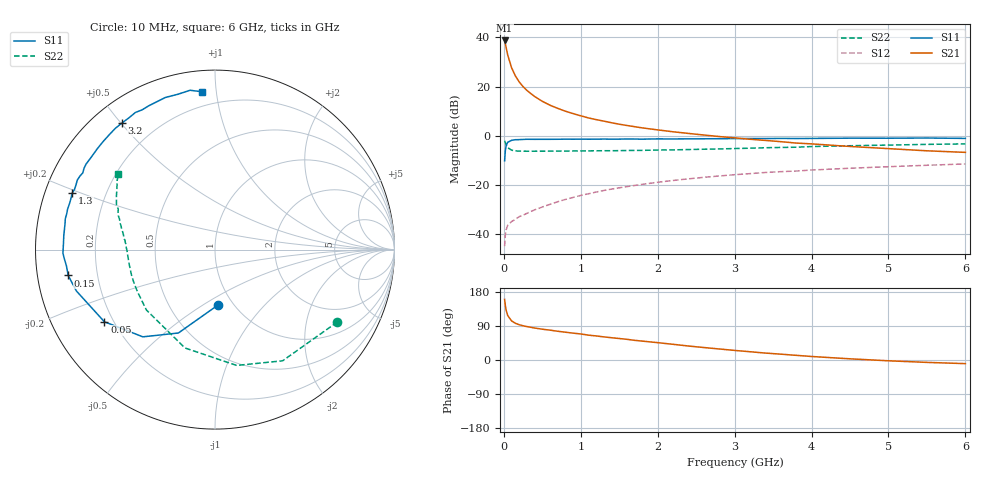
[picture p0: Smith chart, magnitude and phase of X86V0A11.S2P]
! SIEMENS Small Signal Semiconductors
! BFP136W
! Si NPN RF Bipolar Junction Transistor in SOT343
! VCE = 6 V  IC = 110 mA
! Common Emitter S-Parameters:  September  1994
# GHz  S  MA  R  50
!  f  S11  S21  S12  S22
! GHz  MAG  ANG  MAG  ANG  MAG  ANG  MAG  ANG
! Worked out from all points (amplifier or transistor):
!   40 points, 10 MHz to 6 GHz, reference 50 ohm
!   highest |S21| = 38.7 dB at 10 MHz (marker M1)
!   |S21| within 3 dB of that: start of sweep to 30.77 MHz
!   unconditionally stable (mu >= 1): 534.1 MHz to 2.974 GHz
!   at 200 MHz: K = 0.67, MSG = 27.4 dB, |S12| = -32.9 dB
!   at 1.5 GHz: K = 1.10, MAG = 11.0 dB, |S12| = -21.2 dB
!   at 6 GHz: K = 0.97, MSG = 2.4 dB, |S12| = -11.5 dB
!   S11 on the Smith chart (normalised r, x): 10 MHz: 0.85, -0.58; 50 MHz: 0.17, -0.29; 150 MHz: 0.09, -0.09; 1.3 GHz: 0.08, +0.19; 3.2 GHz: 0.08, +0.50; 6 GHz: 0.12, +0.91
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0.01  0.309 -86.8  86.3 159.9  0.0057 69.2  0.7922 -30.6
0.02  0.5075 -113.7  73.61 143.2  0.0099 56.9  0.7251 -58.7
0.03  0.6308 -129.6  61.91 131.5  0.0122 48.1  0.6566 -79.4
0.05  0.7359 -146.9  43.91 117.5  0.0151 38.3  0.573 -107.0
0.1  0.806 -163.4  24.18 103.2  0.018 35.7  0.5092 -138.6
0.15  0.8305 -170.0  16.44 96.9  0.02 38.4  0.4917 -151.6
0.2  0.8327 -173.8  12.37 93.1  0.0227 41.1  0.4875 -158.7
0.25  0.8416 -176.7  9.964 90.3  0.0243 44.3  0.4862 -163.2
0.3  0.8476 -178.7  8.33 88.2  0.0265 46.5  0.4847 -166.2
0.4  0.8449 177.5  6.274 84.4  0.0312 50.9  0.4851 -170.3
0.5  0.8461 174.7  5.003 81.3  0.0356 54.4  0.4855 -173.1
0.6  0.8462 172.7  4.173 78.8  0.0404 56.2  0.4862 -174.9
0.7  0.8481 170.1  3.599 75.8  0.0456 58.0  0.4874 -176.2
0.9  0.85 166.4  2.817 70.9  0.0557 59.5  0.4895 -178.8
1.1  0.8501 162.1  2.302 65.6  0.0662 60.2  0.4926 179.5
1.3  0.8556 158.4  1.979 61.0  0.0772 60.3  0.4955 177.8
1.7  0.8569 151.4  1.526 51.9  0.0977 58.2  0.5028 174.7
2.2  0.8605 143.1  1.204 41.4  0.1232 54.7  0.5159 171.0
3.2  0.8755 126.3  0.848 21.8  0.1697 45.4  0.5578 162.4
4.5  0.8915 108.1  0.605 3.1  0.2185 33.5  0.626 151.3
5.5  0.8986 98.9  0.494 -6.3  0.2512 25.5  0.6672 144.8
6  0.8823 94.7  0.459 -9.6  0.2671 21.3  0.6828 142.0
